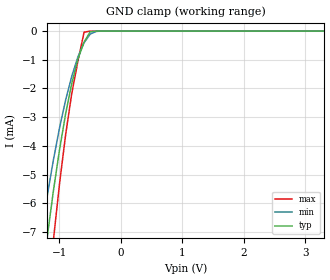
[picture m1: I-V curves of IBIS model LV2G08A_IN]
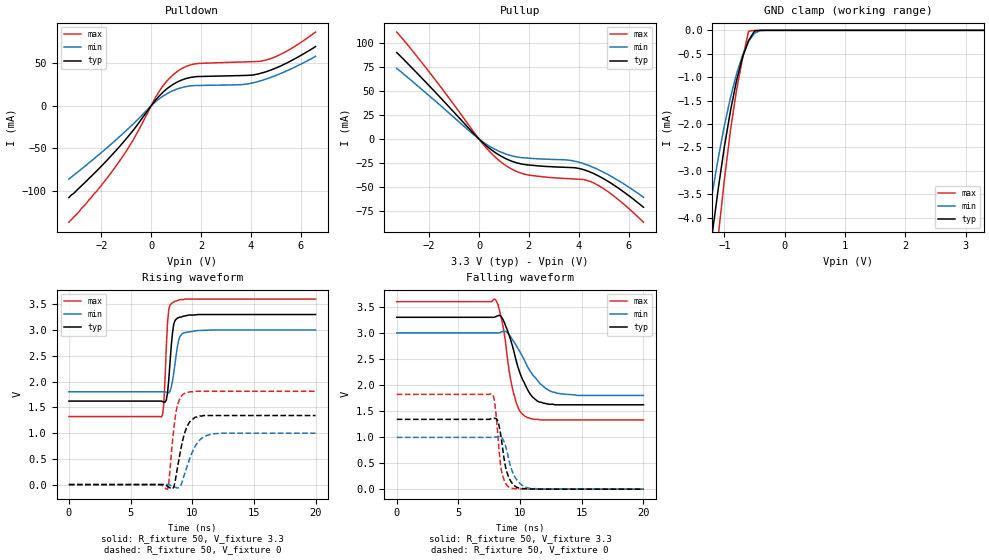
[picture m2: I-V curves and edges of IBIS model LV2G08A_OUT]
|/_/_/_/_/_/_/_/_/_/_/_/_/_/_/_/_/_/_/_/_/_/_/_/_/_/_/_/_/_/_/_/_/_/_/_/_/_/
|   Renesas Electronics Corp.
|   Multi Purpose Semiconductor Digital IC Design Group
|   IBIS Model of HD74LV2G08A
|   3.3V Dual 2-input AND Gates,  SSOP-8(8pin) Package
|   History
|   V1.0   April   1, 2003   : First release.
|/_/_/_/_/_/_/_/_/_/_/_/_/_/_/_/_/_/_/_/_/_/_/_/_/_/_/_/_/_/_/_/_/_/_/_/_/_/
[IBIS Ver]   2.1
[Comment Char]  |_char
[File name]   l2g08s3.ibs
[File Rev]   1.1
[Date]   April 1, 2003
[Source]   Data created from SPICE simulations at
|   Renesas Electronics Corp.
[Notes]   RLC value of the Package is determined by assuming typical
|   conditions.
[Disclaimer]   This information is for modeling purposes only, and is not
|   guaranteed.
[Copyright]   Copyright 2003, Renesas Electronics Corp.,
|   All Rights Reserved.
|   Component  HD74LV2G08A
[Component]   HD74LV2G08A
[Manufacturer]  Renesas Electronics Corp.
[Package]
|   typ   min   max
R_pkg   0.099   0.095   0.102
L_pkg   1.740nH   1.680nH   1.790nH
C_pkg   0.140pF   0.140pF   0.150pF
[Pin]   signal_name   model_name   R_pin   L_pin   C_pin
1   1A   LV2G08A_IN   0.102   1.780nH   0.140pF
2   1B   LV2G08A_IN   0.097   1.710nH   0.150pF
3   2Y   LV2G08A_OUT   0.095   1.680nH   0.150pF
4   GND   GND   0.102   1.790nH   0.140pF
5   2A   LV2G08A_IN   0.101   1.790nH   0.140pF
6   2B   LV2G08A_IN   0.097   1.710nH   0.150pF
7   1Y   LV2G08A_OUT   0.097   1.710nH   0.150pF
8   VCC   POWER   0.102   1.790nH   0.140pF
| Models and submodels in the file (2): LV2G08A_IN (Input), LV2G08A_OUT (Output)
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|   Model  LV2G08A_IN
[Model]   LV2G08A_IN
Model_type  Input
Vinl = 0.99V
Vinh = 2.31V
| variable   typ   min   max
C_comp   2.35pF   2.25pF   2.45pF
| variable   typ   min   max
[Temperature range]   25   85   -40
| variable   typ   min   max
[Voltage range]   3.3V   3.0V   3.6V
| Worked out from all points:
|   GND clamp passes 1 mA (typ) near -0.70 V on its own axis
[GND Clamp]
|   Voltage   I(typ)   I(min)   I(max)
-3.3V     -64mA      -52mA      -81.2mA
-1.3V     -8.95mA    -7.12mA    -11.9mA
-1.2V     -7.19mA    -5.75mA    -9.48mA
-1.1V     -5.58mA    -4.5mA     -7.3mA
-1V       -4.14mA    -3.38mA    -5.33mA
-900mV    -2.88mA    -2.4mA     -3.61mA
-800mV    -1.82mA    -1.57mA    -2.17mA
-700mV    -976uA     -897uA     -1.05mA
-600mV    -380uA     -405uA     -38.6uA
-500mV    -22.3uA    -104uA     -465nA
-400mV    -445nA     -10.5uA    -2.66nA
3.3V      6.7pA      30.3pA     6.6pA
|   Model  LV2G08A_OUT
[Model]   LV2G08A_OUT
Model_type  Output
Polarity   Inverting
Vmeas = 1.65V
| variable   typ   min   max
C_comp   4.85pF   4.75pF   4.95pF
| variable   typ   min   max
[Temperature range]   25   85   -40
| variable   typ   min   max
[Voltage range]   3.3V   3.0V   3.6V
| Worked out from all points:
|   slope of the pulldown table from 0 to 0.495 V, typ, clamps not added: 29.9 ohm
|   slope of the pullup table from 0 to 0.495 V, typ, clamps not added: 44.6 ohm
|   GND clamp passes 1 mA (typ) near -0.78 V on its own axis
|   rising waveform, R_fixture 50, V_fixture 3.3: 20-80 % time 346ps typ, 447ps min, 259ps max; typ from 1.62 V to 3.3 V
|   rising waveform, R_fixture 50, V_fixture 0: 20-80 % time 727ps typ, 1.01ns min, 493ps max; typ from 0 V to 1.34 V
|   falling waveform, R_fixture 50, V_fixture 3.3: 20-80 % time 1.41ns typ, 1.89ns min, 945ps max; typ from 3.3 V to 1.62 V
|   falling waveform, R_fixture 50, V_fixture 0: 20-80 % time 607ps typ, 818ps min, 447ps max; typ from 1.34 V to 0 V
[Pullup]
|   Voltage   I(typ)   I(min)   I(max)
-3.3V     89.7mA     73.3mA     111mA
-1.7V     47.1mA     38.3mA     59.6mA
-47.7nV   3.32pA     32.8pA     3.6pA
500mV     -11.2mA    -8.69mA    -15mA
1V        -19.4mA    -14.8mA    -26.2mA
1.5V      -24.6mA    -18.5mA    -33.6mA
1.9V      -26.7mA    -19.7mA    -36.9mA
3.6V      -29.5mA    -21.9mA    -41.1mA
4V        -30.5mA    -24mA      -41.7mA
4.5V      -34.7mA    -28.5mA    -44.4mA
5.3V      -45.9mA    -38.7mA    -57mA
6.6V      -70.8mA    -60.4mA    -86.3mA
[Pulldown]
|   Voltage   I(typ)   I(min)   I(max)
-3.3V     -108mA     -86.2mA    -137mA
-2.2V     -77.1mA    -60mA      -101mA
-1.3V     -49mA      -37.1mA    -66.4mA
-700mV    -28.1mA    -20.8mA    -39.2mA
300mV     10.8mA     7.71mA     15.9mA
1V        27.3mA     19.4mA     39.4mA
1.5V      32.9mA     23.2mA     47.5mA
1.9V      34.6mA     24mA       50mA
3.7V      35.8mA     25.2mA     51.7mA
4.6V      40.1mA     31.4mA     53.8mA
5.4V      49.8mA     40.7mA     63.7mA
6.6V      69.9mA     58.3mA     86.9mA
[GND Clamp]
|   Voltage   I(typ)   I(min)   I(max)
-3.3V     -38.9mA    -31.6mA    -49.2mA
-1.3V     -5.4mA     -4.31mA    -7.13mA
-1.2V     -4.33mA    -3.47mA    -5.69mA
-1.1V     -3.36mA    -2.71mA    -4.37mA
-1V       -2.48mA    -2.03mA    -3.18mA
-900mV    -1.72mA    -1.44mA    -2.14mA
-800mV    -1.08mA    -936uA     -1.28mA
-700mV    -575uA     -533uA     -610uA
-600mV    -219uA     -237uA     -20.5uA
-500mV    -12.9uA    -58.6uA    -245nA
-400mV    -248nA     -6.13uA    -1.4nA
3.3V      3.42pA     32.9pA     3.3pA
[Ramp]
| variable   typ   min   max
dV/dt_r   0.805/727.1p   0.597/1.006n   1.087/497.5p
dV/dt_f   1.010/1.411n   0.719/1.904n   1.362/942.3p
R_load = 50ohms
[Rising Waveform]
R_fixture = 50
V_fixture = 3.3
V_fixture_min = 3.0
V_fixture_max = 3.6
C_fixture = 0p
|   Time   V(typ)   V(min)   V(max)
0s        1.62V      1.8V       1.32V
7.5ns     1.62V      1.8V       1.31V
7.7ns     1.6V       1.8V       1.58V
8ns       1.78V      1.78V      3.15V
8.1ns     2.04V      1.78V      3.4V
8.4ns     2.94V      2.01V      3.53V
8.6ns     3.18V      2.34V      3.56V
8.9ns     3.24V      2.8V       3.58V
9.4ns     3.27V      2.95V      3.6V
20ns      3.3V       3V         3.6V
[Rising Waveform]
R_fixture = 50
V_fixture = 0
C_fixture = 0p
|   Time   V(typ)   V(min)   V(max)
0s        332pV      676nV      118pV
8ns       -32.8mV    1.8mV      -89.1mV
8.1ns     -49.2mV    -3.14mV    28.8mV
8.4ns     -83.4mV    -31.9mV    838mV
8.7ns     179mV      -59.6mV    1.43V
9.1ns     717mV      -1.46mV    1.71V
9.6ns     1.14V      366mV      1.79V
10.4ns    1.31V      804mV      1.81V
11.4ns    1.34V      969mV      1.81V
20ns      1.34V      997mV      1.81V
[Falling Waveform]
R_fixture = 50
V_fixture = 3.3
V_fixture_min = 3.0
V_fixture_max = 3.6
C_fixture = 0p
|   Time   V(typ)   V(min)   V(max)
0s        3.3V       3V         3.6V
8ns       3.31V      3V         3.64V
8.6ns     3.26V      3.03V      3.14V
9.2ns     2.89V      2.94V      2.14V
9.6ns     2.54V      2.79V      1.73V
10ns      2.22V      2.63V      1.49V
10.6ns    1.91V      2.35V      1.37V
11.4ns    1.69V      2.09V      1.34V
13ns      1.62V      1.84V      1.33V
20ns      1.62V      1.8V       1.33V
[Falling Waveform]
R_fixture = 50
V_fixture = 0
C_fixture = 0p
|   Time   V(typ)   V(min)   V(max)
0s        1.34V      994mV      1.82V
7.7ns     1.35V      995mV      1.83V
8ns       1.36V      1V         1.54V
8.2ns     1.3V       1.01V      1.02V
8.5ns     921mV      994mV      338mV
8.8ns     447mV      843mV      122mV
9.2ns     168mV      457mV      24.2mV
9.9ns     21.6mV     128mV      4.56mV
10.8ns    4mV        16.3mV     341uV
20ns      -21uV      -52.3uV    -4.72uV
